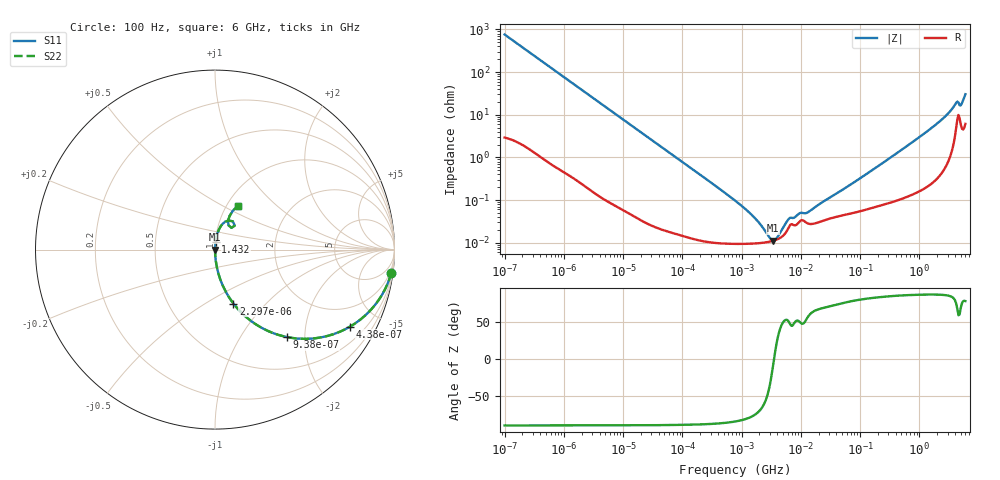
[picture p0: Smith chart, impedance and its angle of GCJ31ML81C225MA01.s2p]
!Murata Part Number: GCJ31ML81C225MA01
!These Parameters are Measured in Series Mode Connection
!Data Generated on Mar 13, 2026
!  o--ll--o
!Port1  Port2
!  o------o
!Operation Temp=25[degC], DC Bias Voltage=0[V]
!Freq. Start=100[Hz] Stop=6[GHz] 401[Steps]
# Hz S RI R 50
!Freq.(Hz) S11(Real) S11(Imag) S21(Real) S21(Imag) S12(Real) S12(Imag) S22(Real) S22(Imag)
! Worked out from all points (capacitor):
!   401 points, 100 Hz to 6 GHz, reference 50 ohm
!   read as one part in series: C = 2.09 uF near 109 Hz
!   lowest |Z| = 11.2 mohm at 3.394 MHz (marker M1)
!   series resonance near 3.533 MHz, so ESL is about 970 pH
!   S11 on the Smith chart (normalised r, x): 100 Hz: 1, -15; 438 Hz: 1.02, -3.50; 938 Hz: 1.01, -1.64; 2.297 kHz: 1.00, -0.67; 1.432 GHz: 1.00, +0.09; 6 GHz: 1.12, +0.59
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100  0.9826 -0.1289  0.0174 0.1289  0.0174 0.1289  0.9826 -0.1289
234  0.9129 -0.2793  0.0871 0.2793  0.0871 0.2793  0.9129 -0.2793
438  0.7522 -0.4291  0.2478 0.4291  0.2478 0.4291  0.7522 -0.4291
656  0.5772 -0.4913  0.4228 0.4913  0.4228 0.4913  0.5772 -0.4913
938  0.4017 -0.4874  0.5983 0.4874  0.5983 0.4874  0.4017 -0.4874
2008  0.1297 -0.3329  0.8703 0.3329  0.8703 0.3329  0.1297 -0.3329
2297  0.1026 -0.3004  0.8974 0.3004  0.8974 0.3004  0.1026 -0.3004
7695  0.0107 -0.0994  0.9893 0.0994  0.9893 0.0994  0.0107 -0.0994
40335  0.000586 -0.0193  0.9994 0.0193  0.9994 0.0193  0.000586 -0.0193
774597  9.44e-05 -0.000968  0.9999 0.000968  0.9999 0.000968  9.44e-05 -0.000968
1658239  9.57e-05 -0.000372  0.9999 0.000372  0.9999 0.000372  9.57e-05 -0.000372
2967816  0.000105 -7.95e-05  0.9999 7.95e-05  0.9999 7.95e-05  0.000105 -7.95e-05
3394479  0.00011 -1.83e-05  0.9999 1.83e-05  0.9999 1.83e-05  0.00011 -1.83e-05
4060267  0.000121 6.47e-05  0.9999 -6.47e-05  0.9999 -6.47e-05  0.000121 6.47e-05
6353432  0.000238 0.000281  0.9998 -0.000281  0.9998 -0.000281  0.000238 0.000281
1.555665e7  0.000275 0.000542  0.9997 -0.000542  0.9997 -0.000542  0.000275 0.000542
3.124326e8  0.00094 0.00941  0.9991 -0.00941  0.9991 -0.00941  0.00094 0.00941
1.431855e9  0.00398 0.0428  0.996 -0.0428  0.996 -0.0428  0.00398 0.0428
2.679998e9  0.0131 0.0868  0.9869 -0.0868  0.9869 -0.0868  0.0131 0.0868
4.009986e9  0.0563 0.1549  0.9437 -0.1549  0.9437 -0.1549  0.0563 0.1549
5.016141e9  0.0752 0.1354  0.9248 -0.1354  0.9248 -0.1354  0.0752 0.1354
6e9  0.1258 0.2441  0.8742 -0.2441  0.8742 -0.2441  0.1258 0.2441
